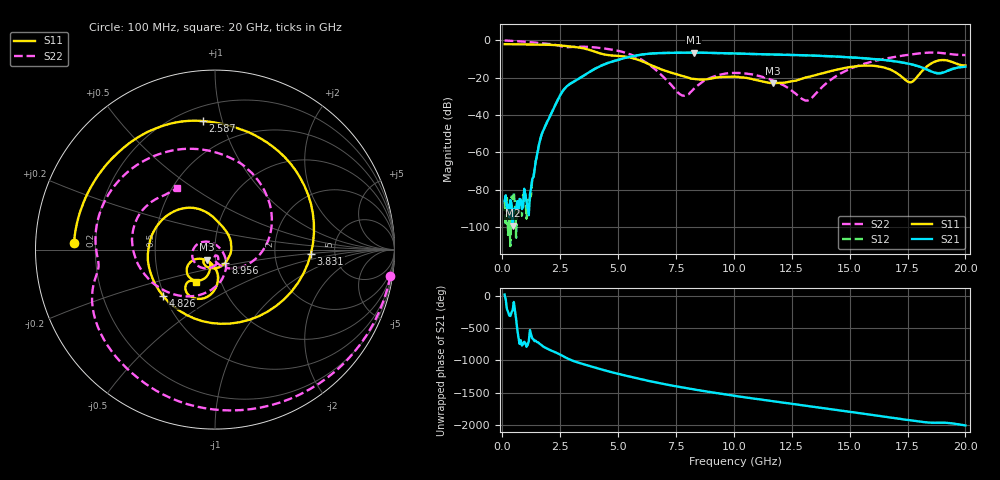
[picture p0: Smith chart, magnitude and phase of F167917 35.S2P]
!  2-Port S-parameters saved by WinCal
! VAR MeasName=S-Parameters (CALIBRATED_DATA) read from VNA (N5242A)
! VAR MeasDate=2016-11-22 9:01:29
! VAR NAME=F167917 35
! VAR FILENAME=F167917 35.S2P
! VAR DATE=2016-11-22 9:01:29
! VAR PHYS_PORTS=1,2
# Hz S DB R 50
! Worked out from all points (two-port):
!   401 points, 100 MHz to 20 GHz, reference 50 ohm
!   highest |S21| = -6.61 dB at 8.259 GHz (marker M1); lowest = -99.3 dB at 448.2 MHz (marker M2)
!   |S21| within 3 dB of the highest: 5.252 GHz to 15.62 GHz (10.37 GHz wide, 99.3 % of centre)
!   lowest |S11| = -22.9 dB at 11.69 GHz (marker M3), VSWR 1.15, Z = 45.5 - j5.09 ohm
!   |S11| at or under -10 dB: 5.749 GHz to end of sweep
!   |S22| runs from -32.3 to -0.1 dB; largest |S21 - S12| = 0.0043
!   S11 on the Smith chart (normalised r, x): 100 MHz: 0.12, +0.02; 2.587 GHz: 0.29, +0.87; 3.831 GHz: 3.29, -0.21; 4.826 GHz: 0.49, -0.30; 8.956 GHz: 1.11, -0.16; 20 GHz: 0.76, -0.29
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1e8  -2.09 177.3  -86.16 20.3  -86.66 27.9  -0.10 -8.7
4.4825e8  -2.13 168.0  -99.28 138.4  -85.12 53.8  -0.33 -36.8
1.24425e9  -2.26 146.2  -79.10 119.4  -82.72 99.0  -1.06 -94.1
1.692e9  -2.35 132.4  -50.71 -41.5  -50.72 -42.0  -1.58 -121.4
2.5875e9  -2.86 95.4  -27.61 154.0  -27.60 153.7  -3.37 -167.5
3.43325e9  -4.14 39.9  -19.58 29.9  -19.60 30.0  -3.44 161.8
3.83125e9  -5.43 -2.4  -16.48 -12.0  -16.47 -11.8  -3.64 142.9
4.32875e9  -7.38 -71.2  -13.32 -63.3  -13.25 -63.2  -4.27 118.3
4.82625e9  -8.23 -138.4  -11.11 -110.9  -11.05 -111.2  -5.25 91.6
5.82125e9  -10.28 134.3  -8.07 164.0  -8.08 163.6  -9.10 25.4
6.7665e9  -15.08 91.5  -6.87 90.3  -6.90 90.1  -17.36 -50.9
7.71175e9  -18.91 51.5  -6.67 26.8  -6.69 26.9  -29.20 -88.9
8.259e9  -20.68 10.3  -6.61 -7.0  -6.62 -6.8  -26.22 -68.1
8.9555e9  -20.63 -51.5  -6.75 -47.7  -6.74 -47.7  -20.28 -97.5
1.005e10  -19.47 -115.6  -7.05 -107.9  -7.04 -107.8  -17.48 -149.6
1.169175e10  -22.94 -128.7  -7.62 168.9  -7.59 168.9  -21.54 149.7
1.338325e10  -19.12 -104.5  -8.18 85.4  -8.16 85.6  -30.64 11.3
1.497525e10  -14.42 -115.8  -9.13 7.4  -9.08 7.2  -15.50 -76.1
1.67165e10  -15.50 -151.2  -10.85 -80.1  -10.91 -80.1  -9.42 -132.4
1.7612e10  -22.53 -120.8  -12.74 -125.9  -12.66 -125.8  -7.64 -160.3
1.875625e10  -11.10 -103.1  -17.66 -163.9  -17.51 -163.7  -6.61 157.4
2e10  -13.46 -120.6  -14.18 154.4  -14.06 154.2  -7.93 121.9
